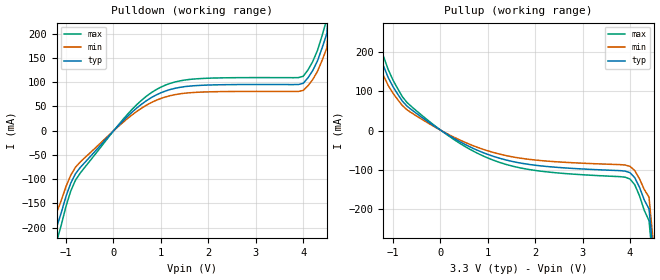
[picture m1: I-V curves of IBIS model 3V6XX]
[IBIS Ver]   2.1
[File name]   55202_3.ibs
[File Rev]   2.0
[Date]   7/20/01
[Source]   ICS MicroClock Applications Engineering 2
[Disclaimer] This information is for modeling purposes only, and is
(C) Copyright Integrated Circuit Systems, Inc. 1997-2001
   All rights reserved
ICS hereby grants the user of this IBIS model a non-exclusive,
nontransferable license to use this IBIS model under the following terms.
Before using this IBIS model, the user should read this license.
If the user does not accept these terms,  the IBIS model should be
returned to ICS within 30 days.
   The user is granted this license only to use the IBIS model and
is not granted rights to sell, load, rent, lease or license the IBIS
model in whole or in part, or in modified form to anyone other than
user. User may modify the IBIS model to suit its specific
applications but rights to derivative works and such modifications
shall belong to ICS.
   This IBIS model is provided on an "AS IS" basis and ICS makes
absolutely no warranty with respect to the information contained
herein. ICS DISCLAIMS AND CUSTOMER WAIVES ALL WARRANTIES, EXPRESS
OR IMPLIED, INCLUDING WARRANTIES OF MERCHANTABILITY OR FITNESS FOR
A PARTICULAR PURPOSE. The entire risk as to quality and performance
is with the Customer. ACCORDINGLY, IN NO EVENT SHALL THE COMPANY BE
LIABLE FOR ANY DAMAGES, WHETHER IN CONTRACT OR TORT,INCLUDING ANY
LOST PROFITS OR OTHER INCIDENTAL, CONSEQUENTIAL, EXEMPLARY, OR
PUNITIVE DAMAGES ARISING OUT OF THE USE OR APPLICATION OF THE IBIS
model provided in this package. Further, ICS reserves the right to
make changes without notice to any product herein to improve
reliability, function, or design. ICS does not convey any license
under patent rights or any other intellectual property rights,
including those of third parties.
   ICS is not obligated to provide maintenance or support
for the licensed IBIS model.
[Component]   ICS552-02
[Manufacturer] Integrated Circuit Systems Inc.
[Package]
|   typ   min   max
R_pkg   40m   35m   45m
L_pkg   1.65nH   1.35nH   1.95nH
C_pkg   0.24pF   0.14pF   0.34pF
[pin]   signal_name   model_name   R_pin   L_pin   C_pin
   3   Q0   3V6XX
   4   Q1   3V6XX
   5   Q2   3V6XX
   6   Q3   3V6XX
 11   Q4   3V6XX
 12   Q5   3V6XX
 13   Q6   3V6XX
 14   Q7   3V6XX
| Models and submodels in the file (1): 3V6XX (Output)
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|   ICS552-02 3.3V Clock Drive Model
| This model is suitable for all output pins on the
|  ICS552-02
[Model]   3V6XX
Model_type   Output
Polarity   Non-Inverting
|   typ   min   max
C_comp   5pF   4pF   6pF
|   typ   min   max
[Voltage range]  3.3V   3.15V   3.45V
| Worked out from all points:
|   slope of the pulldown table from 0 to 0.495 V, typ, clamps not added: 10.4 ohm
|   slope of the pullup table from 0 to 0.495 V, typ, clamps not added: 14 ohm
[pulldown]
|Voltage I (typ)   I (min)   I (max)
-3.3V     -3A        -3A        -3A
-1.2V     -200.1mA   -170mA     -230.1mA
-1.1V     -169.4mA   -144mA     -194.8mA
-900mV    -108.4mA   -92.1mA    -124.6mA
-700mV    -76.24mA   -64.8mA    -87.68mA
400mV     38.57mA    32.79mA    44.36mA
1.1V      81.57mA    69.34mA    93.81mA
1.8V      92.97mA    79.03mA    106.9mA
4V        97.22mA    82.64mA    111.8mA
4.3V      143.1mA    121.7mA    164.6mA
4.5V      200.3mA    170.3mA    230.3mA
6.6V      3A         3A         3A
[pullup]
|Voltage I (typ)   I (min)   I (max)
-3.3V     3A         3A         3A
-1.3V     200.3mA    170.2mA    230.3mA
-1.1V     135.6mA    115.3mA    156mA
-1V       112.4mA    95.55mA    129.3mA
-700mV    61.99mA    52.69mA    71.29mA
200mV     -13.76mA   -11.69mA   -15.82mA
900mV     -56.35mA   -47.89mA   -64.8mA
1.9V      -87.07mA   -74.01mA   -100.1mA
4V        -107.7mA   -91.55mA   -123.9mA
4.1V      -120.5mA   -102.4mA   -138.6mA
4.4V      -200.1mA   -170.1mA   -230.1mA
6.6V      -3A        -3A        -3A
[Ramp]
|   typ   min   max
dV/dt_r   1.56/0.36n   1.48/0.40n   1.64/0.32n
dV/dt_f   1.65/0.32n   1.57/0.35n   1.73/0.29n
